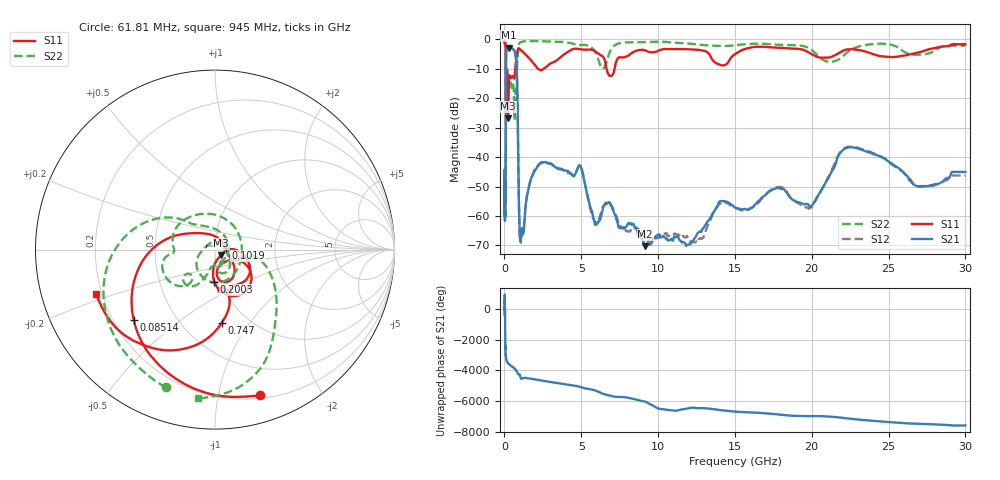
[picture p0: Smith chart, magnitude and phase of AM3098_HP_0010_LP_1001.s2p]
! Date/Time: Thu, Feb 28, 2019 8:33 AM
! Network Analyzer: Agilent Technologies E8364B Rev: A.07.50.67
! Sweep from 0.010 to 30.000 GHz, 1601 Points, Sweep Type: LOG
! Power Supply: 5.022 V, 0.002 A
# Hz S DB R 50
!freq MagS11 AngS11 MagS21 AngS21 MagS12 AngS12 MagS22 AngS22
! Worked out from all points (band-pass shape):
!   1601 points, 10 MHz to 30 GHz, reference 50 ohm
!   highest |S21| = -2.77 dB at 267.8 MHz (marker M1); lowest = -70.2 dB at 9.164 GHz (marker M2)
!   |S21| within 3 dB of the highest: 107.2 MHz to 735 MHz (627.8 MHz wide, 149 % of centre)
!   lowest |S11| = -26.8 dB at 233.9 MHz (marker M3), VSWR 1.10, Z = 53.4 - j3.29 ohm
!   |S11| at or under -10 dB: 92.13 MHz to 701.6 MHz (609.5 MHz wide, 154 % of centre); 2.191 GHz to 2.549 GHz (358 MHz wide, 15.1 % of centre); 6.643 GHz to 7.168 GHz (525.4 MHz wide, 7.61 % of centre)
!   |S22| runs from -27.5 to -0.5 dB; largest |S21 - S12| = 0.011
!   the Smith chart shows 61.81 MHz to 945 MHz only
!   S11 on the Smith chart (normalised r, x): 61.81 MHz: 0.23, -1.33; 85.14 MHz: 0.28, -0.35; 101.9 MHz: 1.13, +0.02; 200.3 MHz: 0.93, -0.35; 747 MHz: 0.76, -0.75; 945 MHz: 0.18, -0.17
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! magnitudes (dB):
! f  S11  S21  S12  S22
! 10 MHz  -0.4  -47.5  -44.6  -0.6
! 38.04 MHz  -0.5  -58.4  -59.5  -1.0
! 61.81 MHz  -1.4  -52.0  -54.1  -1.8
! 75.13 MHz  -2.3  -49.6  -49.2  -2.7
! 85.14 MHz  -4.4  -30.3  -30.1  -4.9
! 101.9 MHz  -24.5  -7.1  -7.1  -17.4
! 144.7 MHz  -15.1  -3.5  -3.4  -13.0
! 200.3 MHz  -14.9  -3.1  -3.1  -10.9
! 233.9 MHz  -26.8  -2.9  -2.8  -12.5
! 267.8 MHz  -17.3  -2.8  -2.7  -12.9
! 550.5 MHz  -12.5  -3.3  -3.3  -14.7
! 747 MHz  -7.7  -6.3  -6.2  -21.1
! 833.9 MHz  -4.2  -15.9  -15.9  -7.6
! 945 MHz  -3.0  -56.3  -58.0  -1.6
! 1.071 GHz  -3.6  -67.6  -66.2  -0.9
! 2.084 GHz  -9.4  -43.8  -43.4  -0.6
! 4.903 GHz  -3.3  -42.8  -42.7  -2.0
! 7.926 GHz  -5.9  -63.5  -64.8  -1.0
! 9.164 GHz  -3.7  -70.2  -67.5  -0.9
! 19.7 GHz  -4.2  -55.8  -57.1  -2.7
! 22.67 GHz  -3.4  -36.7  -36.5  -3.2
! 30 GHz  -1.6  -45.0  -46.2  -2.1
